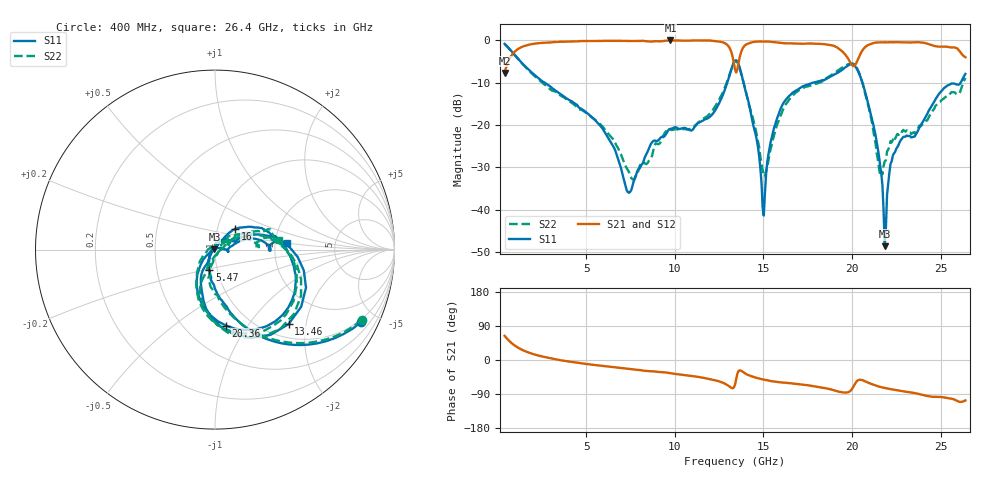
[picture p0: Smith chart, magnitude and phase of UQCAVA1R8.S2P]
!  Part Number  UQCAVA1R8
!  Description: Broardband capacitor  Mounting Orientation: Horizontal
!  Application:
# GHZ S DB R 50
! Freq  |S11|  S11 Ph  |S21|  S21 Ph  |S12|  S12 Ph  |S22|  S22 Ph
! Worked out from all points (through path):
!   401 points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, 400 MHz to 26.4 GHz, reference 50 ohm
!   highest |S21| = -0.01 dB at 9.76 GHz (marker M1); lowest = -7.7 dB at 400 MHz (marker M2)
!   group delay of S21, straight-line fit = 12.9 ps
!   lowest |S11| = -48.6 dB at 21.85 GHz (marker M3), VSWR 1.01, Z = 49.7 + j0.141 ohm
!   |S11| at or under -10 dB: 2.667 GHz to 12.96 GHz (10.29 GHz wide, 132 % of centre); 13.88 GHz to 17.78 GHz (3.902 GHz wide, 24.6 % of centre); 20.59 GHz to 26.13 GHz (5.536 GHz wide, 23.7 % of centre)
!   |S22| runs from -32.9 to -0.9 dB; largest |S21 - S12| = 0.01
!   S11 on the Smith chart (normalised r, x): 400 MHz: 0.88, -4.11; 5.47 GHz: 0.92, -0.21; 13.46 GHz: 1.27, -1.60; 16 GHz: 1.21, +0.29; 20.36 GHz: 0.77, -0.80; 26.4 GHz: 2.32, +0.22
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0.4  -0.82 -26.3  -7.69 63.8  -7.74 63.8  -0.85 -25.6
1.83  -7.20 -70.8  -0.96 18.5  -1.00 18.6  -7.38 -71.4
4.755  -16.22 -98.1  -0.15 -8.8  -0.17 -8.6  -16.44 -101.4
5.47  -18.70 -105.9  -0.14 -13.1  -0.15 -12.9  -18.61 -103.5
7.42  -36.00 137.4  -0.14 -23.6  -0.12 -23.3  -31.11 -63.7
9.11  -23.46 47.2  -0.22 -31.6  -0.19 -31.2  -24.45 39.0
9.76  -20.91 39.3  -0.01 -34.9  -0.01 -34.5  -21.11 37.9
12.815  -11.79 19.2  -0.63 -62.1  -0.61 -62.0  -11.25 16.3
13.4  -4.79 -33.5  -6.82 -65.2  -6.80 -65.2  -4.92 -39.1
13.465  -4.68 -45.3  -7.59 -51.0  -7.56 -50.9  -4.85 -50.6
13.92  -10.70 -102.7  -1.35 -33.8  -1.32 -33.7  -10.52 -104.0
14.635  -23.67 -122.8  -0.28 -47.4  -0.24 -47.4  -22.58 -109.4
14.96  -39.52 -164.9  -0.25 -51.1  -0.22 -51.1  -30.64 -75.1
16  -15.89 45.9  -0.61 -59.2  -0.58 -59.2  -17.51 32.8
17.755  -10.03 17.9  -0.74 -68.6  -0.70 -68.8  -10.50 20.8
19.64  -6.33 -21.1  -3.45 -85.9  -3.42 -86.2  -5.99 -26.0
20.355  -7.38 -81.8  -4.32 -53.1  -4.28 -53.4  -7.18 -84.3
21.33  -22.36 -141.1  -0.52 -67.3  -0.49 -67.6  -24.32 -158.6
21.85  -48.61 157.6  -0.44 -73.8  -0.41 -74.1  -28.59 82.1
22.11  -31.29 18.1  -0.44 -76.1  -0.41 -76.5  -25.21 52.3
22.825  -23.19 -3.6  -0.45 -82.1  -0.42 -82.5  -21.64 26.4
26.4  -7.91 5.6  -3.97 -106.7  -3.94 -107.3  -8.88 8.7
